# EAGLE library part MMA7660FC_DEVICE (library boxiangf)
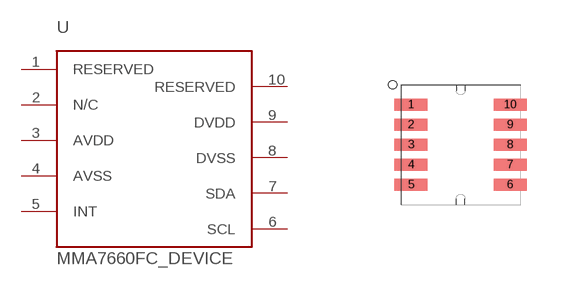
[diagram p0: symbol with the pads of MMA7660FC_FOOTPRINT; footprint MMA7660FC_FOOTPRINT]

Designator prefix -

## MMA7660FC_DEVICE  [MMA7660FC_FOOTPRINT]
1  RESERVED  in
2  N/C  in
3  AVDD  in
4  AVSS  in
5  INT  out
6  SCL  in
7  SDA  oc
8  DVSS  in
9  DVDD  in
10  RESERVED  in

## Footprint MMA7660FC_FOOTPRINT (pad centres in mm)
smd 0.825 x 0.3: 1 -1.24,1; 2 -1.24,0.5; 3 -1.24,0; 4 -1.24,-0.5; 5 -1.24,-1; 6 1.24,-1; 7 1.24,-0.5; 8 1.24,0; 9 1.24,0.5; 10 1.24,1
